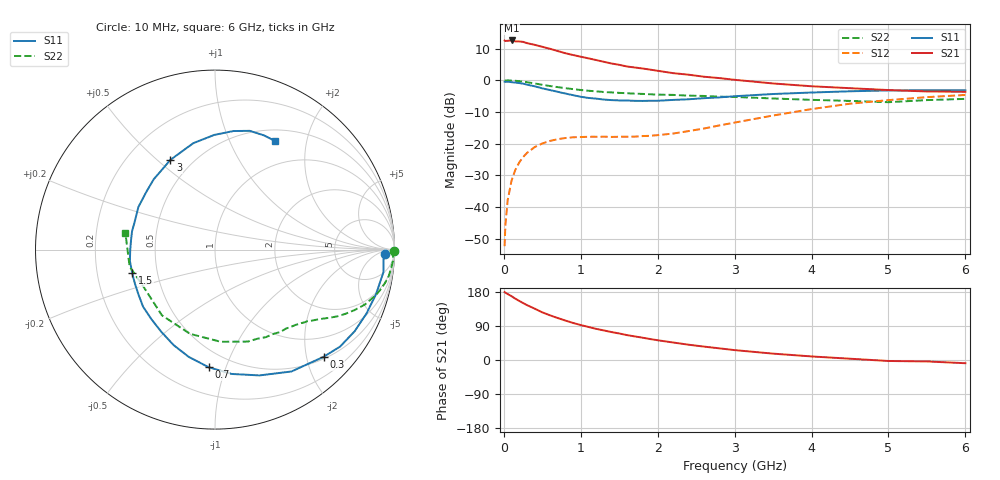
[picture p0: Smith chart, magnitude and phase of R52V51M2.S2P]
! SIEMENS Small Signal Semiconductors
! BFR183
! Si NPN RF Bipolar Junction Transistor in SOT23
! VCE = 2.5 V  IC = 1.2 mA
! Common Emitter S-Parameters:  May  1996
# GHz  S  MA  R  50
!  f  S11  S21  S12  S22
! GHz  MAG  ANG  MAG  ANG  MAG  ANG  MAG  ANG
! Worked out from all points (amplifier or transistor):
!   36 points, 10 MHz to 6 GHz, reference 50 ohm
!   highest |S21| = 12.5 dB at 100 MHz (marker M1)
!   |S21| within 3 dB of that: start of sweep to 652.1 MHz
!   unconditionally stable (mu >= 1): 1.576 GHz to 2.92 GHz
!   at 250 MHz: K = 0.17, MSG = 18.2 dB, |S12| = -24.3 dB
!   at 1.4 GHz: K = 0.91, MSG = 11.6 dB, |S12| = -17.9 dB
!   at 6 GHz: K = 0.95, MSG = 0.5 dB, |S12| = -4.7 dB
!   S11 on the Smith chart (normalised r, x): 10 MHz: 29, -14; 300 MHz: 0.54, -2.33; 700 MHz: 0.38, -0.87; 1.5 GHz: 0.36, -0.12; 3 GHz: 0.38, +0.55; 6 GHz: 0.64, +1.49
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0.01  0.9456 -1.5  4.225 179.2  0.0024 86.5  0.9976 -0.6
0.02  0.9403 -3.0  4.151 177.6  0.0051 91.4  0.9876 -1.1
0.05  0.9471 -7.6  4.191 174.1  0.0128 86.1  0.9959 -2.9
0.1  0.9307 -15.6  4.239 168.4  0.0259 81.5  0.987 -5.8
0.15  0.9161 -22.9  4.1 161.7  0.0386 76.1  0.9794 -8.6
0.2  0.9014 -30.3  4.088 156.0  0.0503 72.3  0.9651 -11.2
0.25  0.8818 -37.8  4.03 150.3  0.0611 68.1  0.9468 -13.8
0.3  0.8505 -44.6  3.85 144.9  0.071 64.5  0.9287 -16.1
0.4  0.8016 -57.9  3.618 135.6  0.0878 57.6  0.8898 -20.1
0.5  0.7436 -70.5  3.366 125.7  0.1003 51.6  0.8464 -23.5
0.7  0.6563 -93.1  2.887 110.8  0.1171 42.8  0.778 -28.5
0.9  0.5804 -113.3  2.497 97.8  0.1256 37.2  0.7229 -32.0
1.1  0.5248 -132.7  2.212 87.2  0.1281 34.2  0.6818 -35.1
1.3  0.4947 -149.4  1.952 78.0  0.1283 33.4  0.6515 -37.7
1.5  0.4794 -164.2  1.748 70.0  0.128 34.4  0.6309 -40.5
1.9  0.4733 167.7  1.47 55.4  0.1326 41.0  0.6001 -46.4
2.2  0.4884 150.9  1.292 46.2  0.1437 46.7  0.586 -51.5
3  0.5582 116.5  1.014 26.1  0.2143 55.6  0.544 -70.4
3.5  0.6053 101.5  0.888 16.8  0.2769 53.7  0.5145 -86.5
4.5  0.6684 81.2  0.748 3.4  0.4257 40.9  0.4708 -128.9
5.5  0.6925 66.7  0.664 -3.8  0.5401 24.5  0.4851 -168.7
6  0.6916 61.2  0.656 -8.5  0.5849 14.6  0.5071 169.7
